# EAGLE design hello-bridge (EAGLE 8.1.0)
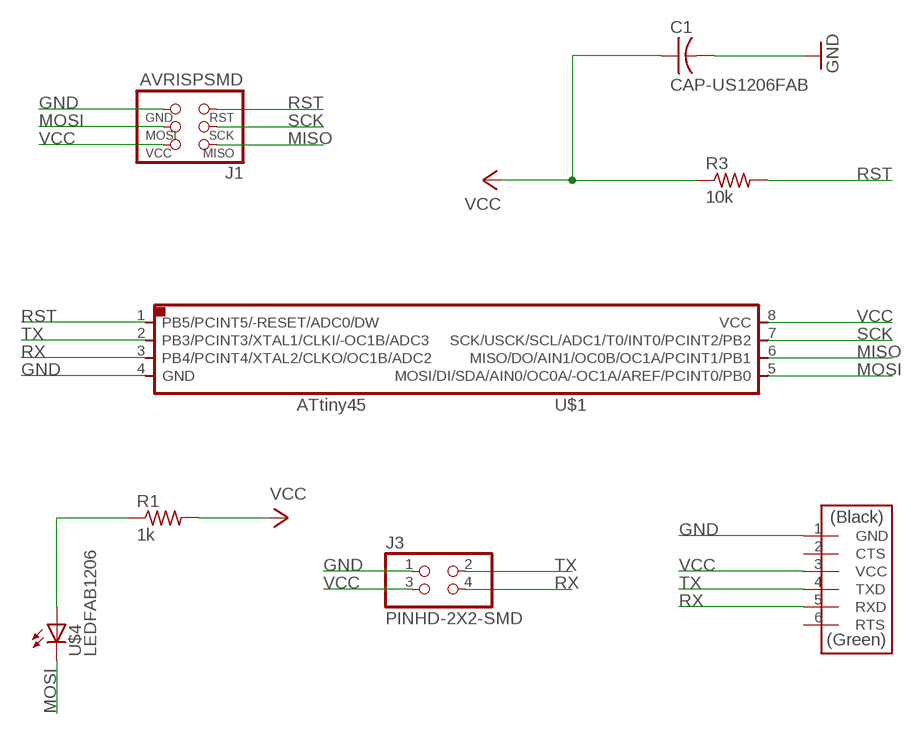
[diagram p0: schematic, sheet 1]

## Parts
C1  CAP-US1206FAB  [C1206FAB]
J1  AVRISPSMD  [2X03SMD]
J3  PINHD-2X2-SMD  [2X02SMD]
R1  1k  RES-US1206FAB  [R1206FAB]
R3  10k  RES-US1206FAB  [R1206FAB]
U$1  ATTINY45SI  [SOIC8]
U$3  FTDI-SMD-HEADER  [1X06SMD]
U$4  LEDFAB1206  [LED1206FAB]

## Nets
GND: C1.2 J1.6(GND) J3.1 U$1.4(GND) U$3.1(GND)
MISO: J1.1(MISO) U$1.6(MISO/DO/AIN1/OC0B/OC1A/PCINT1/PB1)
MOSI: J1.4(MOSI) U$1.5(MOSI/DI/SDA/AIN0/OC0A/-OC1A/AREF/PCINT0/PB0) U$4.2(C)
N$1: R1.1 U$4.1(A)
RST: J1.5(RST) R3.2 U$1.1(PB5/PCINT5/-RESET/ADC0/DW)
RX: J3.4 U$1.3(PB4/PCINT4/XTAL2/CLKO/OC1B/ADC2) U$3.5(RXD)
SCK: J1.3(SCK) U$1.7(SCK/USCK/SCL/ADC1/T0/INT0/PCINT2/PB2)
TX: J3.2 U$1.2(PB3/PCINT3/XTAL1/CLKI/-OC1B/ADC3) U$3.4(TXD)
VCC: C1.1 J1.2(VCC) J3.3 R1.2 R3.1 U$1.8(VCC) U$3.3(VCC)
Unconnected: U$3.2(CTS) U$3.6(RTS)

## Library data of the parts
C1 = 01-fab:CAP-US
J1 = 01-fab:AVRISP
J3 = 01-fab:PINHD-2X2-SMD
R1 R3 = 01-fab:RES-US: Resistor (US Symbol)
U$1 = 01-fab:ATTINY45
U$3 = 01-fab:FTDI-SMD-HEADER
U$4 = 01-fab:LED: LED

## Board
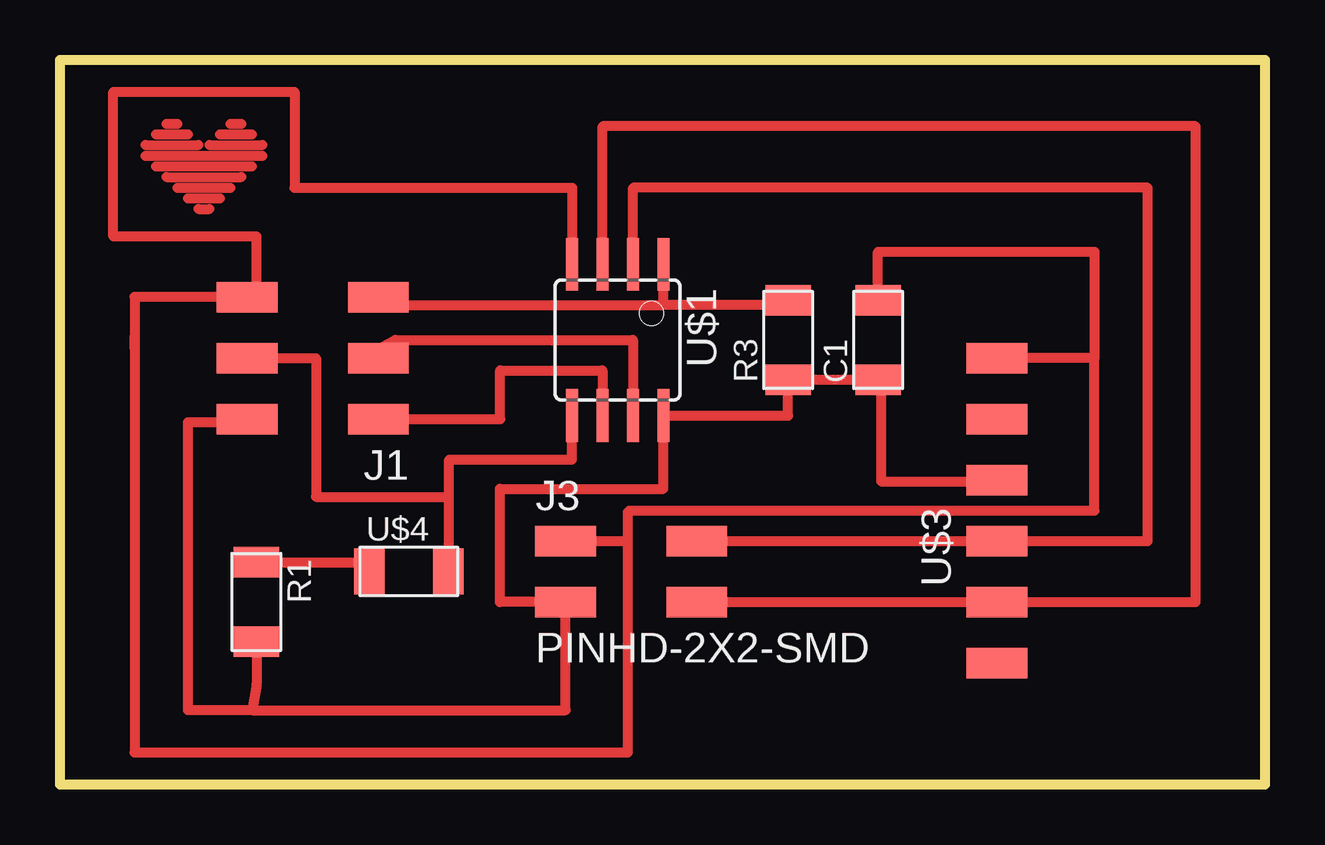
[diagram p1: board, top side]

Size 50.22 x 30.22 mm. Coordinates in mm from the lower left corner, seen from the top.
Outline: 0,0 50.22,0 50.22,30.22 0,30.22 0,0
Copper layers (1*16): Top 0.035mm / dielectric 1.5mm / Bottom 0.035mm
Design rules "default *": minimum track width 10mil, minimum drill 24mil, track to track 16mil, track to pad 16mil, pad to pad 16mil, via to via 16mil, smd to smd 16mil, copper to edge 40mil, drill to drill 8mil, minimum pad ring 10mil, minimum via ring 8mil, stop-mask expansion 4mil, vias tented up to drill 0mil, thermal gap 10mil
Milling: 4 lines

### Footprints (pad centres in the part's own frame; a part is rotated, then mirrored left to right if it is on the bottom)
C1206FAB = smd 1.27 x 1.905: 1 -1.651,0; 2 1.651,0
2X03SMD = smd 2.54 x 1.27: 1 -2.54,2.54; 2 2.92,2.54; 3 -2.54,0; 4 2.92,0; 5 -2.54,-2.54; 6 2.92,-2.54
2X02SMD = smd 2.54 x 1.27: 1 -2.54,1.27; 2 2.92,1.27; 3 -2.54,-1.27; 4 2.92,-1.27
R1206FAB = smd 1.27 x 1.905: 1 -1.651,0; 2 1.651,0
SOIC8 = smd 0.5 x 2.2: 1 -1.905,-3.154; 2 -0.645,-3.154; 3 0.625,-3.154; 4 1.895,-3.154; 5 1.905,3.154; 6 0.635,3.154; 7 -0.635,3.154; 8 -1.905,3.154
1X06SMD = smd 2.54 x 1.27: 1 0,6.35; 2 0,3.81; 3 0,1.27; 4 0,-1.27; 5 0,-3.81; 6 0,-6.35
LED1206FAB = smd 1.27 x 1.905: 1 -1.651,0; 2 1.651,0

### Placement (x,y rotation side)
C1  34.1,18.54 90 top
J1  10.73,17.78 180 top
J3  23.62,8.89 0 top
R1  8.19,7.62 270 top
R3  30.35,18.54 90 top
U$1  23.24,18.54 180 top
U$3  39.05,11.43 0 top
U$4  14.54,8.89 0 top

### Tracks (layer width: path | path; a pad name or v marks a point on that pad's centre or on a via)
GND
  Top 0.406: J1.6 8.19,20.32 8.19,22.86 2.22,22.86 2.22,28.89 9.78,28.89 9.78,24.89 21.35,24.89 U$1.4 | C1.2 34.1,22.23 43.12,22.23 43.12,17.78 | 43.12,17.78 U$3.1 | 7.81,20.34 J1.6 | J1.6 7.8,20.34 3.11,20.34 3.11,18.22 | 23.67,10.22 23.67,11.37 23.73,11.43 43.12,11.43 43.12,17.78 | J3.1 23.61,10.16 23.67,10.22 | 3.11,18.22 3.11,1.33 23.67,1.33 23.67,10.22 | 3.11,18.22 3.11,18.67
MISO
  Top 0.406: J1.1 18.35,15.24 18.35,17.27 22.61,17.27 U$1.6
MOSI
  Top 0.406: J1.4 10.67,17.78 10.67,12 16.19,12 U$4.2 16.22,8.89 16.22,13.56 21.34,13.56 U$1.5
N$1
  Top 0.406: R1.1 12.89,9.27 U$4.1
N$2
  Top 0.406: 4.45,27.56 4.89,27.56
N$3
  Top 0.406: 4,27.11 5.33,27.11
N$4
  Top 0.406: 3.56,26.67 5.78,26.67
N$5
  Top 0.406: 3.56,26.23 8.45,26.23
N$6
  Top 0.406: 7.11,27.56 7.56,27.56
N$7
  Top 0.406: 6.67,27.11 8,27.11
N$8
  Top 0.406: 6.22,26.67 8.45,26.67
N$9
  Top 0.406: 4,25.78 8,25.78
N$10
  Top 0.406: 4.45,25.34 7.56,25.34
N$11
  Top 0.406: 4.89,24.89 7.11,24.89
N$12
  Top 0.406: 5.33,24.45 6.67,24.45
N$13
  Top 0.406: 5.78,24 6.22,24
RST
  Top 0.406: J1.5 13.34,20.32 13.34,20 25.15,20 | R3.2 30.23,20.19 30.23,20 25.15,20 | 25.15,20 U$1.1
RX
  Top 0.406: J3.4 U$3.5 47.34,7.62 47.34,27.45 22.62,27.45 U$1.3
SCK
  Top 0.406: J1.3 12.97,18 13.97,18.54 23.88,18.54 U$1.7
TX
  Top 0.406: J3.2 U$3.4 45.34,10.16 45.34,24.89 23.89,24.89 U$1.2
VCC
  Top 0.406: 38.23,12.67 38.16,12.78 U$3.3 39.05,12.65 34.23,12.65 34.23,16.89 C1.1 R3.1 30.35,15.39 U$1.8 25.15,12.34 18.34,12.34 18.34,7.62 J3.3 21.08,3.11 8,3.11 | J1.2 7.81,15.11 5.33,15.11 5.33,3.11 8,3.11 | R1.2 8.19,4.19 8,3.11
